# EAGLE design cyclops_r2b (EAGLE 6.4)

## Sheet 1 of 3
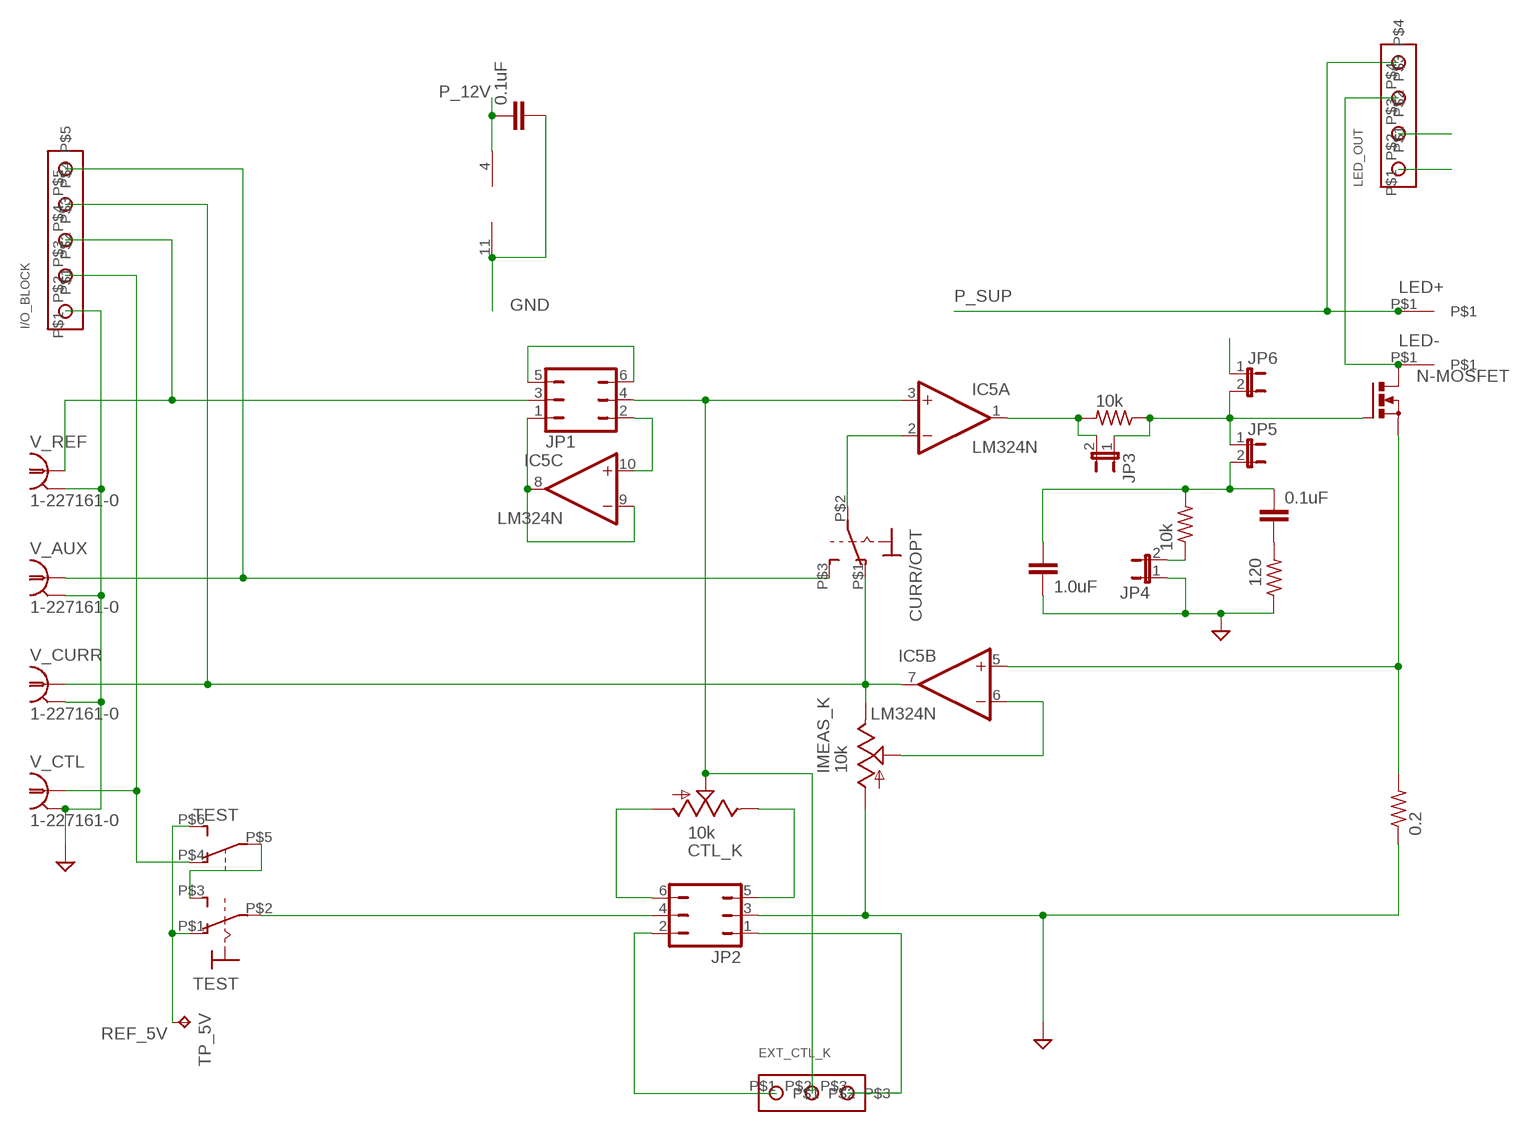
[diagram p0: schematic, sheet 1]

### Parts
C2  0.1uF  C-EU050-024X044  [C050-024X044]
C3  1.0uF  C-EU025-024X044  [C025-024X044]
C7  0.1uF  C-EU050-024X044  [C050-024X044]
CTL_K  10k  TRIM_US-RJ6S  [RJ6S]
CURR/OPT  SPST_SWITCH  [A_TOGGLE_SPST]
EXT_CTL_K  SCREW3  [SCREW3]
I/O_BLOCK  SCREW5  [SCREW5]
IC5  LM324N  [DIL14]
IMEAS_K  10k  TRIM_US-RJ6S  [RJ6S]
JP1  JP3Q  [JP3Q]
JP2  JP3Q  [JP3Q]
JP3  JP1E  [JP1]
JP4  JP1E  [JP1]
JP5  JP1E  [JP1]
JP6  JP1E  [JP1]
LED+  BANANA_TO_BOARD  [BANANA_TO_BOARD]
LED-  BANANA_TO_BOARD  [BANANA_TO_BOARD]
LED_OUT  SCREW4  [SCREW4]
N-MOSFET  PMOSFET_NTO220BH  [TO220BH]
R3  10k  R-US_0207/7  [0207/7]
R4  10k  R-US_0207/7  [0207/7]
R8  120  R-US_0207/7  [0207/7]
R_CURR  0.2  R-US_  [IMEAS_R]
TEST  SP3T_SWITCH  [320-938]
TP_5V  TPPAD1-13  [P1-13]
V_AUX  1-227161-0  [AMP_227161]
V_CTL  1-227161-0  [AMP_227161]
V_CURR  1-227161-0  [AMP_227161]
V_REF  1-227161-0  [AMP_227161]

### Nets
GND: C3.2 C7.2 I/O_BLOCK.P$1 IC5.11(P:V-) IMEAS_K.A JP2.3 JP4.1 LED_OUT.P$1 R8.1 R_CURR.1 V_AUX.2(GND) V_CTL.2(GND) V_CURR.2(GND) V_REF.2(GND) ; also sheet 2,3
N$1: CURR/OPT.P$2(P) IC5.2(A:-IN)
N$2: IC5.5(B:+IN) N-MOSFET.S R_CURR.2
N$3: IC5.1(A:OUT) JP3.2 R4.2
N$4: CURR/OPT.P$1(O) I/O_BLOCK.P$4 IC5.7(B:OUT) IMEAS_K.E V_CURR.1
N$5: CURR/OPT.P$3(S) I/O_BLOCK.P$5 V_AUX.1
N$6: JP2.4 TEST.P$2(1:P)
N$7: CTL_K.E JP2.5
N$8: CTL_K.S EXT_CTL_K.P$2 IC5.3(A:+IN) JP1.4
N$9: IC5.8(C:OUT) IC5.9(C:-IN) JP1.1
N$10: I/O_BLOCK.P$2 TEST.P$4(B:O) V_CTL.1
N$11: C2.1 C3.1 JP5.2 R3.2
N$12: CTL_K.A JP2.6
N$13: C2.2 R8.2
N$14: IC5.10(C:+IN) JP1.2
N$15: IC5.6(B:-IN) IMEAS_K.S
N$17: JP1.5 JP1.6
N$18: I/O_BLOCK.P$3 JP1.3 V_REF.1
N$21: LED-.P$1 LED_OUT.P$3 N-MOSFET.D
N$23: TEST.P$3(1:S) TEST.P$5(B:P)
N$25: EXT_CTL_K.P$1 JP2.2
N$26: EXT_CTL_K.P$3 JP2.1
N$27: JP4.2 R3.1
N$29: JP3.1 JP5.1 JP6.2 N-MOSFET.G R4.1
N$69: JP6.1
P_12V: C7.1 IC5.4(P:V+) LED_OUT.P$2 ; also sheet 2
P_SUP: LED+.P$1 LED_OUT.P$4 ; also sheet 2,3
REF_5V: TEST.P$1(1:O) TEST.P$6(B:S) TP_5V.TP ; also sheet 2
Unconnected: IC5.12(D:+IN) IC5.13(D:-IN) IC5.14(D:OUT)

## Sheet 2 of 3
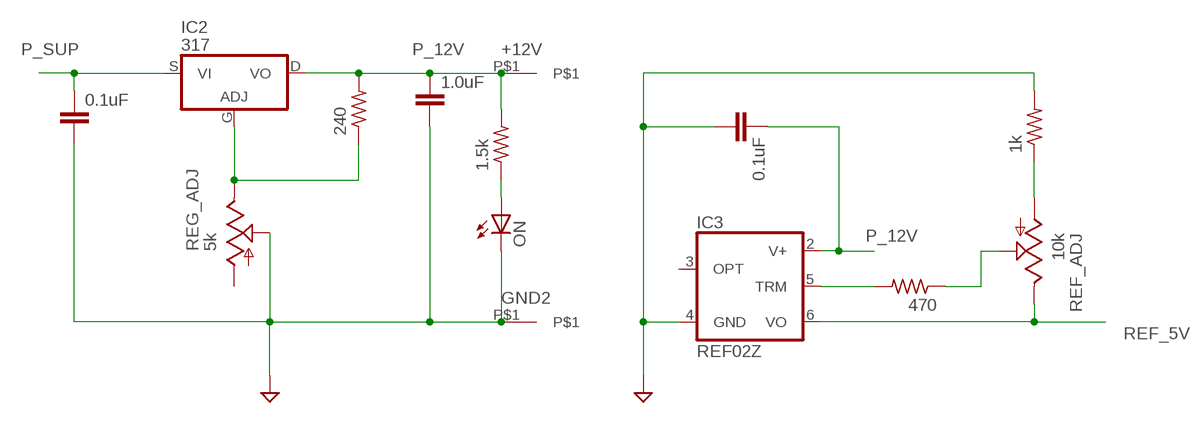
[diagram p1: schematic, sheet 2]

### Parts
+12V  BANANA_TO_BOARD  [BANANA_TO_BOARD]
C4  0.1uF  C-EU050-024X044  [C050-024X044]
C5  1.0uF  C-EU025-024X044  [C025-024X044]
C6  0.1uF  C-EU050-024X044  [C050-024X044]
GND2  BANANA_TO_BOARD  [BANANA_TO_BOARD]
IC2  317  [TO220BH]
IC3  REF02Z  [DIL08]
ON  LED3MM  [LED3MM]
R2  1.5k  R-US_0207/7  [0207/7]
R9  1k  R-US_0207/7  [0207/7]
R10  240  R-US_0207/7  [0207/7]
R12  470  R-US_0207/7  [0207/7]
REF_ADJ  10k  TRIM_US-RJ6S  [RJ6S]
REG_ADJ  5k  TRIM_US-RJ6S  [RJ6S]

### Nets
GND: C4.2 C5.2 C6.2 GND2.P$1 IC3.4(GND) ON.K(C) R9.2 REG_ADJ.S ; also sheet 1,3
N$19: IC2.G(ADJ) R10.1 REG_ADJ.E
N$20: IC3.5(TRM) R12.2
N$22: R12.1 REF_ADJ.S
N$24: R9.1 REF_ADJ.A
N$28: ON.A R2.1
P_12V: +12V.P$1 C5.1 C6.1 IC2.D(VO) IC3.2(V+) R2.2 R10.2 ; also sheet 1
P_SUP: C4.1 IC2.S(VI) ; also sheet 1,3
REF_5V: IC3.6(VO) REF_ADJ.E ; also sheet 1
Unconnected: IC3.3(OPT) REG_ADJ.A

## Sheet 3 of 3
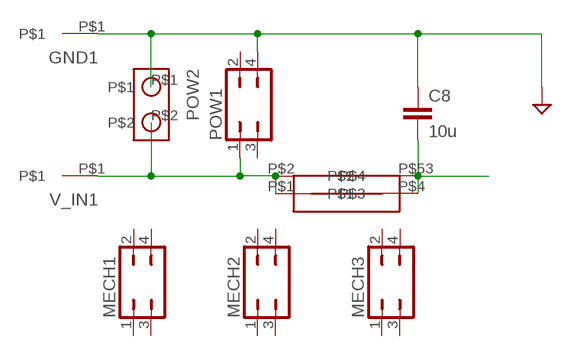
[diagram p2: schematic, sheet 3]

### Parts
C8  10u  C-EU025-024X044  [C025-024X044]
GND1  BANANA_TO_BOARD  [BANANA_TO_BOARD]
MECH1  JP2Q  [JP2Q]
MECH2  JP2Q  [JP2Q]
MECH3  JP2Q  [JP2Q]
POW1  JP2Q  [JP2Q]
POW2  SCREW2  [SCREW2]
U$1  FUSE >2A  NXT-FUSE  [NXT-FUSE]
V_IN1  BANANA_TO_BOARD  [BANANA_TO_BOARD]

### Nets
GND: C8.1 GND1.P$1 POW1.4 POW2.P$1 ; also sheet 1,2
P_SUP: C8.2 U$1.P$4 U$1.P$53 ; also sheet 1,2
P_SUP_BEFORE: POW1.1 POW2.P$2 U$1.P$1 U$1.P$2 V_IN1.P$1
Unconnected: MECH1.1 MECH1.2 MECH1.3 MECH1.4 MECH2.1 MECH2.2 MECH2.3 MECH2.4 MECH3.1 MECH3.2 MECH3.3 MECH3.4 POW1.2 POW1.3

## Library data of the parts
+12V GND1 GND2 LED+ LED- V_IN1 = HOSS:BANANA_TO_BOARD: Female banana socket to board, right angle.
C2-C8 = rcl:C-EU: CAPACITOR, European symbol
CTL_K IMEAS_K REF_ADJ REG_ADJ = HOSS:TRIM_US-: POTENTIOMETER
CURR/OPT = HOSS:SPST_SWITCH: TOGGLE SWITCH distributor RS Components
EXT_CTL_K = HOSS:SCREW3
I/O_BLOCK = HOSS:SCREW5
IC2 = HOSS:*317: Positive VOLTAGE REGULATOR
IC3 = linear:REF02: VOLTAGE REFERENCE
IC5 = linear:LM324: OP AMP
JP1 JP2 = jumper:JP3Q: JUMPER
JP3-JP6 = jumper:JP1E: JUMPER
LED_OUT = HOSS:SCREW4
MECH1-MECH3 POW1 = jumper:JP2Q: JUMPER
N-MOSFET = transistor-power:PMOSFET_N: Power MOSFET N-Channel
ON = led:LED: LED
POW2 = HOSS:SCREW2
R2-R4 R8-R10 R12 R_CURR = HOSS:R-US_: RESISTOR, American symbol
TEST = HOSS:SP3T_SWITCH: TOGGLE SWITCH distributor RS Components
TP_5V = testpad:TP: Test pad
U$1 = HOSS:NXT-FUSE
V_AUX V_CTL V_CURR V_REF = con-coax:?227161*: JACK, RIGHT ANGLE, 50 OHM, PCB, BNC

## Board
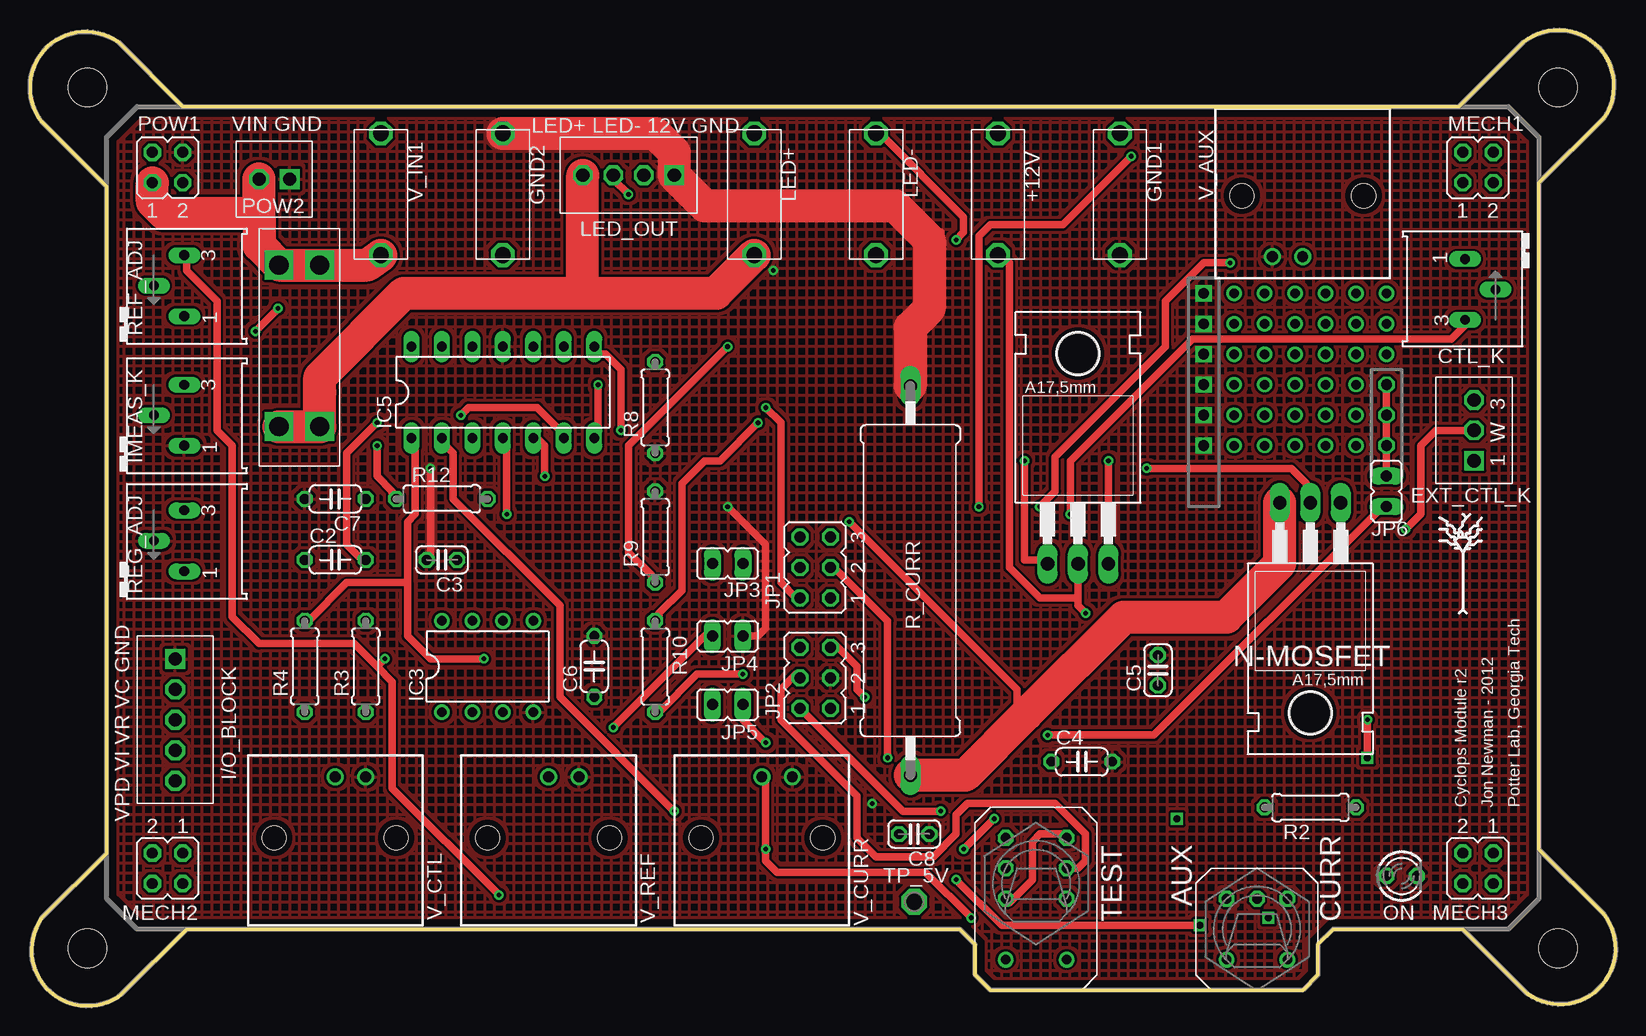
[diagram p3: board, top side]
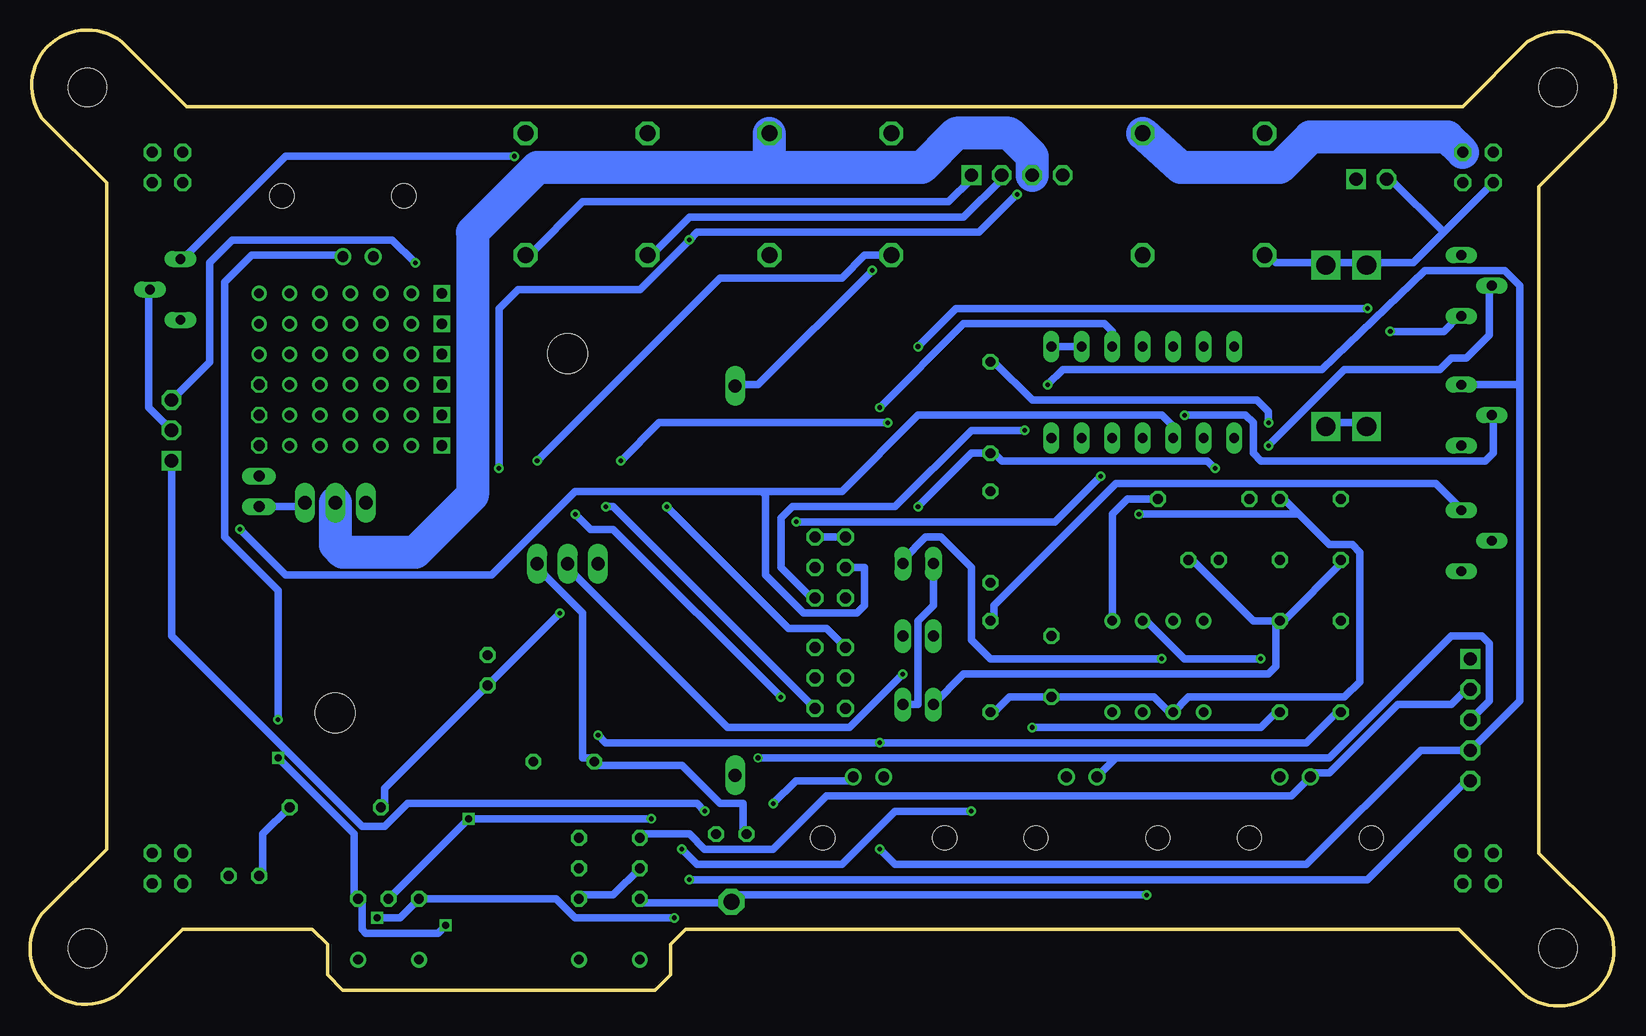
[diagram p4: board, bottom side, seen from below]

Size 132.17 x 81.37 mm. Coordinates in mm from the lower left corner, seen from the top.
Outline: 6.4,12.75 6.4,68.31 1,73.71 arc-164 7.35,80.37 12.75,74.98 119.11,74.98 124.51,80.37 arc-164 131.17,74.02 125.78,68.63 125.78,13.06 131.17,7.67 arc-164 124.82,1 119.43,6.4 108.63,6.4 107.36,5.13 107.36,2.59 106.09,1.32 80.06,1.32 78.79,2.59 78.79,5.13 77.52,6.4 13.06,6.4 7.67,1 arc-164 1,7.35 6.4,12.75
Copper layers (1*16): Top 0.035mm / dielectric 1.5mm / Bottom 0.035mm
Design rules "default *": minimum track width 24mil, minimum drill 15mil, track to track 8mil, track to pad 8mil, pad to pad 8mil, via to via 8mil, smd to smd 8mil, copper to edge 20mil, drill to drill 8mil, minimum pad ring 10mil, minimum via ring 8mil, stop-mask expansion 4mil, vias tented up to drill 0mil, thermal gap 10mil
Holes 3.2 mm at 127.36,76.56 4.81,4.81 127.36,4.81 4.81,76.56
tKeepout: area 77.8,41 to 96.9,58.8; area 97.2,20 to 116.3,37.8

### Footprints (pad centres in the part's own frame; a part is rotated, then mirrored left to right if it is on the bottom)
BANANA_TO_BOARD = drill 1.321 octagon: P$1 0,0; P$2 10.16,0
C050-024X044 = drill 0.813 octagon: 1 -2.54,0; 2 2.54,0
C025-024X044 = drill 0.813 octagon: 1 -1.27,0; 2 1.27,0
RJ6S = drill 0.813 long: A 2.54,-0.2; E -2.54,-0.2; S 0,-2.74
A_TOGGLE_SPST = drill 0.8 octagon: P$1 -2.54,6.35; P$2 0,6.35; P$3 2.54,6.35 | drill 0.8: P$14 2.54,1.27; P$15 -2.54,1.27
SCREW3 = drill 1.1 square: P$1 0,0 | drill 1.1 octagon: P$2 2.54,0; P$3 5.08,0
SCREW5 = drill 1.1 square: P$1 0,0 | drill 1.1 octagon: P$2 2.54,0; P$3 5.08,0; P$4 7.62,0; P$5 10.16,0
TO220BH = drill 1.118 long: D 0,-6.35; G -2.54,-6.35; S 2.54,-6.35 | hole 3.302: 0,11.176
DIL08 = drill 0.813 pad 1.27: 1 -3.81,-3.81; 2 -1.27,-3.81; 3 1.27,-3.81; 4 3.81,-3.81; 5 3.81,3.81; 6 1.27,3.81; 7 -1.27,3.81; 8 -3.81,3.81
DIL14 = drill 0.813 long: 1 -7.62,-3.81; 2 -5.08,-3.81; 3 -2.54,-3.81; 4 0,-3.81; 5 2.54,-3.81; 6 5.08,-3.81; 7 7.62,-3.81; 8 7.62,3.81; 9 5.08,3.81; 10 2.54,3.81; 11 0,3.81; 12 -2.54,3.81; 13 -5.08,3.81; 14 -7.62,3.81
JP3Q = drill 0.914 octagon: 1 -2.54,-1.27; 2 -2.54,1.27; 3 0,-1.27; 4 0,1.27; 5 2.54,-1.27; 6 2.54,1.27
JP1 = drill 0.914 long: 1 0,-1.27; 2 0,1.27
SCREW4 = drill 1.1 square: P$1 0,0 | drill 1.1 octagon: P$2 2.54,0; P$3 5.08,0; P$4 7.62,0
JP2Q = drill 0.914 octagon: 1 -1.27,-1.27; 2 -1.27,1.27; 3 1.27,-1.27; 4 1.27,1.27
LED3MM = drill 0.813 octagon: A -1.27,0; K 1.27,0
SCREW2 = drill 1.1 square: P$1 0,0 | drill 1.1 octagon: P$2 2.54,0
0207/7 = drill 0.813 octagon: 1 -3.81,0; 2 3.81,0
IMEAS_R = drill 1.1 long: 1 -3.23,0; 2 29.23,0
320-938 = drill 0.8 octagon: P$1 2.54,3.81; P$2 2.54,1.27; P$3 2.54,-1.27; P$4 -2.54,3.81; P$5 -2.54,1.27; P$6 -2.54,-1.27 | drill 0.8: P$14 2.54,-6.35; P$15 -2.54,-6.35
P1-13 = drill 1.321 pad 2.159 octagon: TP 0,0
NXT-FUSE = drill 1.6 square: P$1 3.048,1.651; P$2 3.048,5.055; P$4 16.51,5.055; P$53 16.51,1.651
AMP_227161 = drill 0.9 pad 1.27: 1 0,-5.08; 2 -2.54,-5.08 | hole 2: -5.08,0; 5.08,0

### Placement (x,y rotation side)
+12V  80.69,62.59 90 top
C2  25.45,37.19 0 top
C3  34.34,37.19 180 top
C4  87.68,20.37 0 top
C5  94.03,27.99 90 top
C6  47.04,28.3 90 top
C7  25.45,42.27 180 top
C8  73.71,14.33 180 top
CTL_K  119.43,59.74 90 top
CURR/OPT  102.28,2.59 0 top
EXT_CTL_K  120.38,45.45 90 top
GND1  90.85,62.59 90 top
GND2  39.42,72.75 270 top
I/O_BLOCK  12.11,28.94 270 top
IC2  87.36,43.23 0 top
IC3  38.15,28.3 0 top
IC5  39.42,51.16 0 top
IMEAS_K  13.06,49.26 270 top
JP1  65.45,36.56 90 top
JP2  65.45,27.35 90 top
JP3  58.15,36.88 270 top
JP4  58.15,30.84 90 top
JP5  58.15,25.13 90 top
JP6  113.08,42.91 180 top
LED+  60.37,62.59 90 top
LED-  70.53,72.75 270 top
LED_OUT  53.7,69.26 180 top
MECH1  120.7,69.9 0 top
MECH2  11.48,11.48 180 top
MECH3  120.7,11.48 180 top
N-MOSFET  106.73,35.61 180 top
ON  114.35,10.84 0 top
POW1  11.48,69.9 0 top
POW2  21.64,68.94 180 top
R2  106.73,16.56 180 top
R3  27.99,28.3 90 top
R4  22.91,28.3 90 top
R8  52.12,49.89 90 top
R9  52.12,39.1 90 top
R10  52.12,28.3 270 top
R12  34.34,42.27 0 top
R_CURR  73.39,48.46 270 top
REF_ADJ  13.06,60.05 270 top
REG_ADJ  13.06,38.78 270 top
TEST  83.87,10.21 0 top
TP_5V  73.71,8.68 0 top
U$1  19.1,64.82 270 top
V_AUX  106.09,67.55 0 top
V_CTL  25.45,14.02 180 top
V_CURR  61.01,14.02 180 top
V_IN1  29.26,62.59 90 top
V_REF  43.23,14.02 180 top

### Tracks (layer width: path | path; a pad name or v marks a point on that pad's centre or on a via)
GND  (via drill 0.38, 0.9)
  Top 0.61: 74.98,63.86 75.93,64.5 | v33.38,44.81 33.38,37.19 C3.2 | v58.15,41.64 61.32,38.46 61.32,31.48 60.69,30.84 JP4.1
  Top 2.769: R_CURR.1 73.39,56.56 74.98,58.15 74.98,63.86 72.12,66.72 56.24,66.72 LED_OUT.P$1 53.7,71.17 52.12,72.75 GND2.P$1
  Bottom 0.61: LED_OUT.P$1 53.7,68.94 55.61,67.04 86.09,67.04 90.53,62.59 GND1.P$1 | v61.96,61.32 71.48,51.8 73.39,51.8 R_CURR.1 | v70.21,16.87 68.31,18.78 63.86,18.78 V_CURR.2 | v33.38,44.81 34.02,45.45 51.16,45.45 51.8,46.08 R8.1 53.7,46.08 v58.15,41.64
  Bottom 2.769: GND2.P$1 36.24,69.9 27.99,69.9 25.45,72.44 14.02,72.44 POW1.4
  other vias: 97.84,46.72 97.84,49.26 97.84,51.8 97.84,54.34 97.84,56.88 97.84,59.42
  pour Top (hatched): 7.35,72.12 9.25,74.02 122.92,74.02 124.82,72.12 124.82,9.25 122.92,7.35 108.31,7.35 106.41,5.44 106.41,2.9 105.77,2.27 80.37,2.27 79.74,2.9 79.74,5.44 77.83,7.35 9.25,7.35 7.35,9.25
N$1  (via drill 0.38, 0.6)
  Top 0.61: v77.83,13.06 v80.37,15.6 | v53.7,16.24 44.18,25.76 44.18,33.38 35.29,42.27 35.29,46.08 34.65,46.72 34.65,47.35 IC5.2
  Bottom 0.61: v80.37,15.6 v95.61,15.6 CURR/OPT.P$2 | v77.83,13.06 76.56,11.79 64.5,11.79 60.05,16.24 v53.7,16.24
N$2  (via drill 0.38)
  Top 0.61: v42.91,44.18 42.91,46.72 42.27,47.35 IC5.5 | v68.31,40.37 82.28,26.4 82.28,25.13 83.07,24.33
  Top 2.769: N-MOSFET.S 104.19,36.88 99.74,32.43 91.17,32.43 83.07,24.33 77.97,19.23 R_CURR.2
  Bottom 0.61: v42.91,44.18 46.72,40.37 v68.31,40.37
N$3  (via drill 0.38)
  Top 0.61: R4.2 23.22,32.11 26.4,35.29 31.48,35.29 | IC5.1 32.11,47.35 32.11,41 31.48,40.37 31.48,35.29 | v37.83,28.94 33.38,28.94 31.48,30.84 31.48,35.29
  Bottom 0.61: JP3.2 59.42,37.19 57.51,39.1 56.24,39.1 53.7,36.56 53.7,30.53 52.12,28.94 v37.83,28.94
N$4  (via drill 0.38, 0.6)
  Top 0.61: v78.47,7.35 74.66,11.16 62.28,11.16 61.32,12.11 v61.32,13.06 61.32,18.78 V_CURR.1 | v47.35,51.8 47.35,47.35 IC5.7
  Bottom 0.61: v47.35,51.8 46.08,53.07 24.49,53.07 15.92,61.32 9.25,61.32 7.98,60.05 7.98,51.8 | v61.32,13.06 60.05,11.79 25.76,11.79 16.24,21.32 I/O_BLOCK.P$4 7.98,25.45 7.98,51.8 | 7.98,51.8 IMEAS_K.E | v103.23,7.35 101.33,7.35 CURR/OPT.P$1 88.31,8.94 86.72,7.35 v78.47,7.35
N$5  (via drill 0.38, 0.6)
  Top 0.61: v111.49,20.68 v111.49,23.86 | v77.2,10.52 81.01,6.71 v97.52,6.71
  Bottom 0.61: v77.2,10.52 20.68,10.52 12.43,18.78 I/O_BLOCK.P$5 | V_AUX.1 106.22,62.59 113.71,62.59 115.93,60.37 115.93,39.1 111.49,34.65 v111.49,23.86 | v97.52,6.71 98.15,6.08 104.19,6.08 104.5,6.4 104.5,8.62 CURR/OPT.P$3 105.14,9.25 105.14,14.33 v111.49,20.68
N$6
  Top 0.61: JP2.4 63.86,27.67 62.59,26.4 62.59,23.86 68.94,17.51 68.94,14.02 70.53,12.43 75.29,12.43 77.2,14.33 77.2,15.92 78.15,16.87 85.45,16.87 87.99,14.33 87.99,12.11 87.36,11.48 TEST.P$2
N$7  (via drill 0.38)
  Top 0.61: v86.72,41 86.72,45.45 96.88,55.61 118.47,55.61 119.63,56.76 CTL_K.E | v69.58,25.76 68.94,26.4 68.94,28.3 67.04,30.21 JP2.5
  Bottom 0.61: v69.58,25.76 83.55,39.73 85.45,39.73 v86.72,41
N$8  (via drill 0.38)
  Top 0.61: v114.66,39.73 115.93,41 115.93,46.72 117.2,47.99 EXT_CTL_K.P$2
  Bottom 0.61: CTL_K.S 122.28,59.42 122.28,49.89 EXT_CTL_K.P$2 | JP1.4 62.59,36.56 62.59,33.38 63.23,32.75 67.67,32.75 70.85,35.92 70.85,42.59 71.17,42.91 | v114.66,39.73 110.85,35.92 93.71,35.92 86.72,42.91 71.17,42.91 | 71.17,42.91 64.5,42.91 58.15,49.26 37.83,49.26 36.88,48.31 IC5.3
N$9  (via drill 0.38)
  Top 0.61: v49.26,47.99 49.26,53.07 47.99,54.34 47.35,54.34 47.35,54.97 IC5.8
  Bottom 0.61: IC5.9 IC5.8 | v49.26,47.99 53.7,47.99 60.05,41.64 68.63,41.64 69.58,40.69 69.58,36.56 67.04,34.02 JP1.1
N$10
  Bottom 0.61: TEST.P$4 81.01,14.33 77.2,14.33 75.93,13.06 70.21,13.06 65.77,17.51 27.03,17.51 V_CTL.1 25.13,19.41 23.86,19.41 18.14,25.13 13.7,25.13 12.43,26.4 I/O_BLOCK.P$2
N$11
  Bottom 0.61: C2.1 22.59,37.19 27.67,32.11 R3.2 28.3,32.11 | 28.3,32.11 30.21,32.11 35.29,37.19 C3.1 | JP5.2 54.34,27.67 28.94,27.67 28.3,28.3 28.3,32.11
N$12  (via drill 0.38)
  Top 0.61: v91.8,70.85 86.09,65.13 80.06,65.13 79.1,64.18 v79.1,41.64
  Bottom 0.61: v91.8,70.85 110.85,70.85 119.11,62.59 CTL_K.A | v79.1,41.64 68.94,31.48 65.77,31.48 JP2.6
N$13  (via drill 0.38)
  Top 0.61: v28.94,48.62 26.4,46.08 26.4,38.46 27.67,37.19 C2.2
  Bottom 0.61: R8.2 51.8,53.7 48.62,50.53 29.89,50.53 28.94,49.58 v28.94,48.62
N$14  (via drill 0.38)
  Top 0.61: v61.32,49.89 62.59,48.62 62.59,35.29 63.86,34.02 JP1.2
  Bottom 0.61: v61.32,49.89 54.34,56.88 42.59,56.88 41.96,56.24 IC5.10
N$15  (via drill 0.38)
  Top 0.61: v35.92,49.26 36.56,49.89 42.27,49.89 44.18,47.99 44.18,47.35 IC5.6
  Bottom 0.61: 10.52,49.26 IMEAS_K.S 10.21,49.14 10.21,46.08 10.84,45.45 29.57,45.45 30.21,46.08 30.21,48.62 30.84,49.26 v35.92,49.26
N$17
  Bottom 0.61: JP1.6 JP1.5
N$18  (via drill 0.38)
  Top 0.61: v71.48,20.68 71.48,32.11 67.04,36.56 JP1.3
  Bottom 0.61: 41.64,20.68 23.86,20.68 13.7,30.84 11.16,30.84 10.52,30.21 10.52,25.45 I/O_BLOCK.P$3 | 41.64,20.68 V_REF.1 | 41.64,20.68 v71.48,20.68
N$19  (via drill 0.38)
  Top 0.61: v82.91,45.45 82.91,37.19 84.82,37.19 IC2.G | v60.69,48.62 57.51,45.45 56.24,45.45 54.34,43.54 54.34,34.65 52.43,32.75 52.43,32.11 R10.1
  Bottom 0.61: v82.91,45.45 79.74,48.62 v60.69,48.62 | REG_ADJ.E 13.06,41.64 14.97,43.54 41.64,43.54 51.8,33.38 51.8,32.11 R10.1
N$20
  Bottom 0.61: 41.64,32.11 IC3.5 41.96,41 40.69,42.27 R12.2
N$21  (via drill 0.38)
  Top 0.61: v49.89,67.67 48.62,68.94 LED_OUT.P$3 | v77.2,63.86 77.83,64.5 77.83,65.77 70.85,72.75 LED-.P$1 | v93.07,44.81 105.14,44.81 106.41,43.54 106.41,42.27 N-MOSFET.D
  Bottom 0.61: v49.89,67.67 53.07,64.5 76.56,64.5 v77.2,63.86 81.33,59.74 91.49,59.74 93.07,58.15 v93.07,44.81
  Bottom 2.769: N-MOSFET.D 106.73,38.46 106.09,37.83 100.06,37.83 95.3,42.59 95.3,64.5 89.9,69.9 70.53,69.9 | LED_OUT.P$3 48.62,70.85 50.53,72.75 54.97,72.75 57.83,69.9 70.53,69.9 | 70.53,69.9 LED-.P$1
N$22  (via drill 0.38)
  Top 0.61: v28.94,46.72 28.94,44.18 30.21,42.91 30.21,42.27 R12.1
  Bottom 0.61: v28.94,46.72 22.59,53.07 14.65,53.07 13.7,54.02 12.43,54.02 10.52,55.93 10.52,59.85 REF_ADJ.S 10.52,60.05
N$23
  Bottom 0.61: TEST.P$5 83.55,9.25 86.09,9.25 TEST.P$3
N$24  (via drill 0.38)
  Top 0.61: v18.78,56.24 v20.68,58.15 | v58.15,54.97 49.89,46.72 49.89,37.83 51.8,35.92 51.8,35.29 R9.1
  Bottom 0.61: v18.78,56.24 14.33,56.24 13.06,57.51 REF_ADJ.A | v20.68,58.15 54.97,58.15 v58.15,54.97
N$25  (via drill 0.38)
  Top 0.61: v75.93,16.24 72.75,16.24 JP2.2
  Bottom 0.61: v75.93,16.24 76.56,16.87 100.69,16.87 102.6,14.97 104.5,14.97 120.38,30.84 EXT_CTL_K.P$1
N$26  (via drill 0.38)
  Top 0.61: v84.18,41.64 85.45,42.91 85.45,45.77 94.66,54.97 94.66,58.78 97.84,61.96 v100.06,61.96
  Bottom 0.61: v84.18,41.64 83.55,41.64 JP2.1 | v100.06,61.96 101.96,63.86 115.3,63.86 117.2,61.96 117.2,53.7 EXT_CTL_K.P$3
N$27  (via drill 0.38)
  Top 0.61: v48.62,23.22 56.24,30.84 JP4.2
  Bottom 0.61: v48.62,23.22 29.57,23.22 28.3,24.49 R3.1
N$28
  Bottom 0.61: ON.A 112.76,11.16 112.76,14.33 R2.1 110.85,16.24
N$29  (via drill 0.38)
  Top 0.61: v84.82,22.59 93.71,22.59 112.76,41.64 JP6.2 | v61.32,21.95 59.42,23.86 JP5.1
  Bottom 0.61: JP6.2 109.58,41.64 N-MOSFET.G | v84.82,22.59 84.18,21.95 v61.32,21.95 25.76,21.95 23.22,24.49 R4.1 | JP5.1 58.15,25.13 58.15,32.11 56.88,33.38 JP3.1
N$32  (via drill 0.8 pad 1.27)
  other vias: 100.38,56.88
N$33  (via drill 0.8 pad 1.27)
  other vias: 113.08,54.34
N$34  (via drill 0.8 pad 1.27)
  other vias: 113.08,56.88
N$35  (via drill 0.8 pad 1.27)
  other vias: 110.54,56.88
N$36  (via drill 0.8 pad 1.27)
  other vias: 108,56.88
N$37  (via drill 0.8 pad 1.27)
  other vias: 105.46,56.88
N$38  (via drill 0.8 pad 1.27)
  other vias: 102.92,56.88
N$39  (via drill 0.8 pad 1.27)
  other vias: 105.46,46.72
N$40  (via drill 0.8 pad 1.27)
  other vias: 100.38,59.42
N$41  (via drill 0.8 pad 1.27)
  other vias: 102.92,59.42
N$42  (via drill 0.8 pad 1.27)
  other vias: 100.38,54.34
N$43  (via drill 0.8 pad 1.27)
  other vias: 102.92,54.34
N$44  (via drill 0.8 pad 1.27)
  other vias: 105.46,54.34
N$45  (via drill 0.8 pad 1.27)
  other vias: 108,54.34
N$46  (via drill 0.8 pad 1.27)
  other vias: 110.54,54.34
N$47  (via drill 0.8 pad 1.27)
  other vias: 110.54,51.8
N$48  (via drill 0.8 pad 1.27)
  other vias: 108,51.8
N$49  (via drill 0.8 pad 1.27)
  other vias: 105.46,51.8
N$50  (via drill 0.8 pad 1.27)
  other vias: 102.92,51.8
N$51  (via drill 0.8 pad 1.27)
  other vias: 100.38,51.8
N$52  (via drill 0.8 pad 1.27)
  other vias: 105.46,59.42
N$53  (via drill 0.8 pad 1.27)
  other vias: 108,59.42
N$54  (via drill 0.8 pad 1.27)
  other vias: 100.38,49.26
N$55  (via drill 0.8 pad 1.27)
  other vias: 102.92,49.26
N$56  (via drill 0.8 pad 1.27)
  other vias: 105.46,49.26
N$57  (via drill 0.8 pad 1.27)
  other vias: 108,49.26
N$58  (via drill 0.8 pad 1.27)
  other vias: 110.54,49.26
N$59  (via drill 0.8 pad 1.27)
  other vias: 110.54,46.72
N$60  (via drill 0.8 pad 1.27)
  other vias: 108,46.72
N$62  (via drill 0.8 pad 1.27)
  other vias: 102.92,46.72
N$63  (via drill 0.8 pad 1.27)
  other vias: 100.38,46.72
N$64  (via drill 0.8 pad 1.27)
  other vias: 110.54,59.42
N$65  (via drill 0.8 pad 1.27)
  other vias: 113.08,59.42
N$69  (via drill 0.9)
  Top 0.61: v113.08,51.8 v113.08,49.26 v113.08,46.72 JP6.1
P_12V  (via drill 0.38)
  Top 0.61: v39.73,41 39.73,47.35 IC5.4 | v87.99,32.75 87.36,33.38 87.36,34.02 | IC2.D 87.36,34.02 | 87.36,34.02 84.18,34.02 81.64,36.56 81.64,61.96 81.01,62.59 +12V.P$1 | v59.42,27.67 55.61,27.67 52.43,24.49 R10.2
  Bottom 0.61: LED_OUT.P$2 51.16,68.94 54.34,65.77 77.2,65.77 80.37,62.59 +12V.P$1 | R2.2 102.6,16.87 102.6,18.14 C5.1 v87.99,32.75 | R10.2 51.8,24.49 50.53,25.76 C6.1 38.46,25.76 37.19,24.49 IC3.2 35.61,25.76 22.59,25.76 21.32,27.03 21.32,37.83 21.95,38.46 23.86,38.46 26.4,41 | 26.4,41 27.67,42.27 C7.1 | 26.4,41 v39.73,41 | v59.42,27.67 63.86,23.22 74.02,23.22 87.36,36.56 IC2.D
P_SUP  (via drill 0.38)
  Top 0.61: v89.9,45.45 IC2.S | 57.2,59.42 57.51,59.1 | 24.15,51.16 24.49,51.16 24.18,52.43
  Top 2.769: LED+.P$1 57.2,59.42 46.08,59.42 | 46.08,59.42 LED_OUT.P$4 | 46.08,59.42 31.16,59.42 24.18,52.43 | 24.15,52.41 24.15,51.16 U$1.P$4 U$1.P$53
  Bottom 0.61: C8.2 72.75,14.33 72.75,16.87 74.66,16.87 77.83,20.05 84.82,20.05 C4.1 85.45,20.68 86.09,20.68 86.09,32.75 89.9,36.56 IC2.S | U$1.P$53 21.32,48.62 23.86,48.62 U$1.P$4 | v89.9,45.45 74.66,60.69 64.5,60.69 62.59,62.59 LED+.P$1
P_SUP_BEFORE
  Top 2.769: 19.1,65.77 19.1,63.42 U$1.P$1 28.11,61.77 V_IN1.P$1 | 19.1,65.77 POW2.P$2 | POW1.1 10.21,67.04 11.16,66.09 18.78,66.09 19.1,65.77
  Bottom 0.61: V_IN1.P$1 28.94,62.59 28.3,61.96 24.49,61.96 U$1.P$2 23.86,61.96 21.32,61.96 U$1.P$1 20.68,61.96 16.87,61.96 14.33,64.5 | POW1.1 14.33,64.5 | 14.33,64.5 18.78,68.94 POW2.P$2
REF_5V  (via drill 0.38)
  Top 0.61: TEST.P$6 81.64,8.62 83.55,10.52 83.55,13.7 84.18,14.33 86.09,14.33 TEST.P$1 | REF_ADJ.E 13.06,62.59 13.06,61.32 15.6,58.78 15.6,47.99 16.87,46.72 16.87,32.43 19.1,30.21 27.03,30.21 28.94,28.3 | v39.1,9.25 30.21,18.14 30.21,27.03 28.94,28.3 | 28.94,28.3 v29.57,28.94
  Bottom 0.61: TEST.P$6 81.01,8.62 74.02,8.62 TP_5V.TP 73.39,9.25 v39.1,9.25 | v29.57,28.94 35.92,28.94 39.1,32.11 IC3.6

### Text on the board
tPlace: VIN GND | LED+ LED- 12V GND | 1 W 3 | VPD VI VR VC GND | AUX | CURR
tNames: Cyclops Module r2 | Jon Newman - 2012 | Potter Lab, Georgia Tech
tDocu: V_GATE | GND | + | + | + | +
